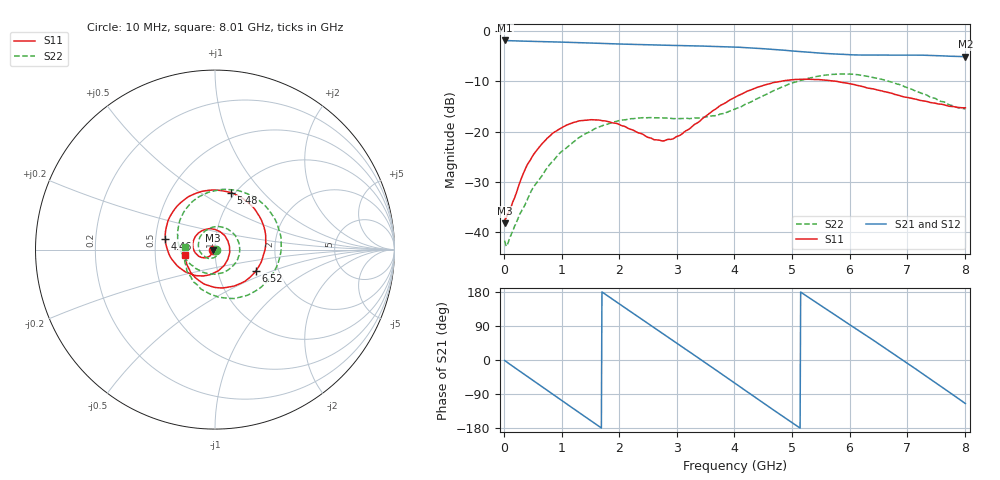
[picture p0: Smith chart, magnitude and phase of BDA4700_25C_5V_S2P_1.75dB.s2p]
!Agilent Technologies,E5071B,MY42404982,A.09.10
!Date: Mon Oct 20 13:26:47 2025
!Data & Calibration Information:
!Freq	S11:SOLT2(ON)	S21:SOLT2(ON)	S12:SOLT2(ON)	S22:SOLT2(ON)
# Hz S RI R 50
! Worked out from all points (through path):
!   801 points, 10 MHz to 8.01 GHz, reference 50 ohm
!   highest |S21| = -1.87 dB at 20 MHz (marker M1); lowest = -5.1 dB at 8.01 GHz (marker M2)
!   group delay of S21, straight-line fit = 288 ps
!   lowest |S11| = -38.2 dB at 10 MHz (marker M3), VSWR 1.02, Z = 48.8 - j0.195 ohm
!   |S11| at or under -10 dB: start of sweep to 4.801 GHz; 5.78 GHz to end of sweep
!   |S22| runs from -42.7 to -8.5 dB; largest |S21 - S12| = 0.0061
!   S11 on the Smith chart (normalised r, x): 10 MHz: 0.98, -0.00; 4.46 GHz: 0.56, +0.07; 5.48 GHz: 0.96, +0.68; 6.52 GHz: 1.54, -0.38; 8.01 GHz: 0.71, -0.05
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1e7  -0.0121 -0.002  0.8061 -0.017  0.806 -0.0184  0.00822 -0.00111
2e7  -0.0131 -0.00341  0.8057 -0.0316  0.8051 -0.0341  0.00795 3.09e-06
3.4e8  -0.0241 -0.0308  0.6372 -0.474  0.6367 -0.4751  0.0159 -0.00793
7.2e8  -0.0694 -0.0448  0.1752 -0.7639  0.1753 -0.764  0.000671 -0.0415
1.02e9  -0.1097 -0.0181  -0.2497 -0.7337  -0.2503 -0.7346  -0.0461 -0.0456
1.35e9  -0.1223 0.041  -0.616 -0.4539  -0.6167 -0.454  -0.0905 0.00708
1.93e9  -0.0366 0.1159  -0.6789 0.3089  -0.679 0.3094  -0.00817 0.1255
2.32e9  0.0414 0.0886  -0.3099 0.6654  -0.3097 0.6658  0.1032 0.0893
2.68e9  0.08 0.021  0.1557 0.7092  0.1558 0.7092  0.1364 -0.0193
3.36e9  0.00912 -0.1223  0.7059 0.0846  0.7065 0.084  -0.00819 -0.1365
3.67e9  -0.0816 -0.1461  0.6332 -0.3041  0.6332 -0.3054  -0.0869 -0.1156
4.01e9  -0.1935 -0.1053  0.3308 -0.6081  0.3315 -0.6078  -0.1559 -0.0618
4.46e9  -0.2767 0.0596  -0.2169 -0.6338  -0.2176 -0.6349  -0.2085 0.0754
4.91e9  -0.1945 0.2586  -0.586 -0.26  -0.5861 -0.2626  -0.1358 0.2577
5.35e9  0.0201 0.3307  -0.5712 0.2214  -0.5719 0.2201  0.0897 0.3333
5.48e9  0.0901 0.3164  -0.4989 0.3411  -0.5 0.3408  0.1654 0.3173
6e9  0.2736 0.1245  -0.0333 0.5813  -0.0355 0.5824  0.3648 0.0819
6.52e9  0.2291 -0.1168  0.4351 0.3806  0.4362 0.3795  0.2721 -0.1948
6.68e9  0.1772 -0.1693  0.5237 0.2415  0.5252 0.2408  0.2022 -0.2435
7.05e9  0.0344 -0.2138  0.5611 -0.1341  0.5614 -0.1362  0.0288 -0.2662
7.45e9  -0.096 -0.1676  0.3227 -0.4721  0.3221 -0.4736  -0.115 -0.1843
8.01e9  -0.1696 -0.0325  -0.2344 -0.5036  -0.2343 -0.5044  -0.168 0.0146
